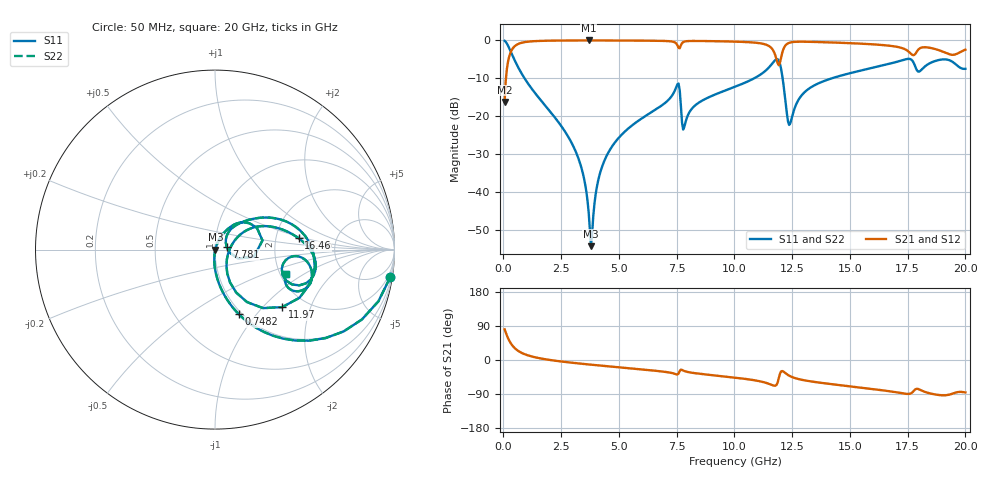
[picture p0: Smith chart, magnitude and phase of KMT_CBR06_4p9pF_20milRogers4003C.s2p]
! Data measured by Modelithics Inc. support@modelithics.com 813-866-6335
! KEMET CBR0603 4.9pF, Pad Width= 0.851mm, Pad Length= 0.64mm, Pad Gap= 0.62mm, 20mil Rogers 4003C substrate Data, January 2022
# hz S ma R 50
! 2 Port Network Data from SP1.SP block
! freq  magS11  angS11  magS21  angS21  magS12  angS12  magS22  angS22
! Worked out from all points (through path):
!   401 points, 50 MHz to 20 GHz, reference 50 ohm
!   highest |S21| = -0.02 dB at 3.691 GHz (marker M1); lowest = -16.3 dB at 50 MHz (marker M2)
!   group delay of S21, straight-line fit = 15.5 ps
!   lowest |S11| = -54.3 dB at 3.791 GHz (marker M3), VSWR 1.00, Z = 50.2 - j0.0612 ohm
!   |S11| at or under -10 dB: 912.4 MHz to 10.86 GHz (9.947 GHz wide, 169 % of centre); 12.09 GHz to 14.22 GHz (2.136 GHz wide, 16.2 % of centre)
!   |S22| runs from -54.3 to -0.1 dB; largest |S21 - S12| = 0
!   S11 on the Smith chart (normalised r, x): 50 MHz: 1, -13; 748.2 MHz: 0.97, -0.81; 7.781 GHz: 1.14, +0.04; 11.97 GHz: 1.53, -1.30; 16.46 GHz: 2.69, +0.44; 20 GHz: 2.16, -0.73
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5e7  0.9881 -9.0  0.1534 81.0  0.1534 81.0  0.9881 -9.0
2.99375e8  0.7301 -44.0  0.6825 45.9  0.6825 45.9  0.7301 -44.0
7.4825e8  0.3827 -69.8  0.9229 20.1  0.9229 20.1  0.3827 -69.8
2.74325e9  0.05742 -94.0  0.9966 -5.7  0.9966 -5.7  0.05742 -94.0
3.391625e9  0.01997 -94.7  0.9979 -9.9  0.9979 -9.9  0.01997 -94.7
3.690875e9  0.005299 -80.9  0.998 -11.8  0.998 -11.8  0.005299 -80.9
3.790625e9  0.001922 -18.5  0.998 -12.4  0.998 -12.4  0.001922 -18.5
4.13975e9  0.01584 68.3  0.9977 -14.4  0.9977 -14.4  0.01584 68.3
4.588625e9  0.03509 69.5  0.9971 -17.0  0.9971 -17.0  0.03509 69.5
6.73325e9  0.1306 58.8  0.9871 -29.4  0.9871 -29.4  0.1306 58.8
7.53125e9  0.2632 27.6  0.8629 -38.3  0.8629 -38.3  0.2632 27.6
7.780625e9  0.06641 14.0  0.9492 -27.8  0.9492 -27.8  0.06641 14.0
1.0025e10  0.2445 42.0  0.9631 -46.5  0.9631 -46.5  0.2445 42.0
1.147138e10  0.4324 20.7  0.8506 -62.3  0.8506 -62.3  0.4324 20.7
1.177062e10  0.5508 -2.6  0.6351 -67.9  0.6351 -67.9  0.5508 -2.6
1.197012e10  0.4927 -40.6  0.5075 -36.4  0.5075 -36.4  0.4927 -40.6
1.236912e10  0.07654 -18.8  0.9285 -41.4  0.9285 -41.4  0.07654 -18.8
1.336662e10  0.2458 29.9  0.9558 -57.0  0.9558 -57.0  0.2458 29.9
1.645888e10  0.4702 7.7  0.8659 -80.3  0.8659 -80.3  0.4702 7.7
1.670825e10  0.4909 5.2  0.8507 -82.4  0.8507 -82.4  0.4909 5.2
1.775562e10  0.5099 -23.0  0.6372 -82.2  0.6372 -82.2  0.5099 -23.0
2e10  0.4215 -19.2  0.7535 -85.7  0.7535 -85.7  0.4215 -19.2
